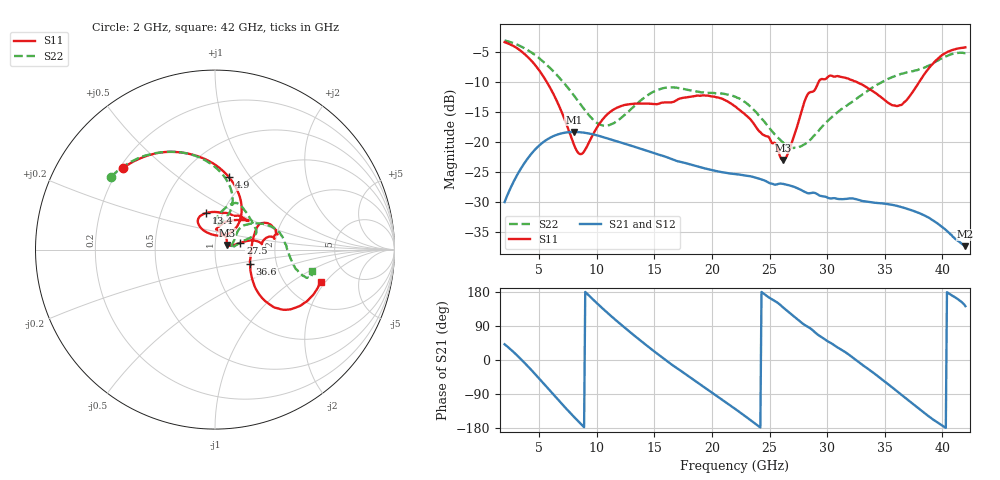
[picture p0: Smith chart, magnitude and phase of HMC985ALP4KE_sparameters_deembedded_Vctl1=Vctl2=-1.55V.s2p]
!s2p File: Measurements: S11, S21, S12, S22
# GHz S dB R 50.0
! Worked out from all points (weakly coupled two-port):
!   401 points, 2 GHz to 42 GHz, reference 50 ohm
!   highest |S21| = -18.30 dB at 8 GHz (marker M1); lowest = -37.4 dB at 42 GHz (marker M2)
!   lowest |S11| = -23.0 dB at 26.2 GHz (marker M3), VSWR 1.15, Z = 57 + j2.93 ohm
!   |S11| at or under -10 dB: 5.678 GHz to 29.25 GHz (23.57 GHz wide, 135 % of centre); 32.61 GHz to 37.97 GHz (5.359 GHz wide, 15.2 % of centre)
!   |S22| runs from -21.0 to -3.0 dB; largest |S21 - S12| = 0.00014
!   S11 on the Smith chart (normalised r, x): 2 GHz: 0.21, +0.36; 4.9 GHz: 0.82, +0.80; 13.4 GHz: 0.84, +0.36; 27.5 GHz: 1.33, +0.10; 36.6 GHz: 1.46, -0.24; 42 GHz: 3.08, -1.83
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2  -3.29 138.5  -30.03 41.5  -30.03 41.5  -3.01 145.0
3.4  -4.75 110.4  -24.48 2.7  -24.48 2.7  -3.98 121.8
4.9  -7.74 79.0  -20.75 -45.6  -20.76 -45.6  -5.82 98.1
6.2  -11.81 54.8  -19.03 -89.9  -19.04 -90.0  -8.10 80.6
8  -20.32 57.3  -18.30 -149.4  -18.31 -149.4  -12.16 68.4
8.7  -21.97 88.8  -18.38 -171.2  -18.39 -171.2  -13.97 69.5
10.8  -15.57 123.2  -19.30 127.9  -19.30 127.9  -17.25 88.6
13.4  -13.56 103.5  -20.86 61.0  -20.87 61.0  -13.72 82.0
15.4  -13.57 77.2  -22.11 13.3  -22.11 13.3  -11.19 68.9
18.9  -12.25 41.7  -24.16 -62.7  -24.16 -62.7  -11.61 42.8
22  -14.01 55.7  -25.35 -128.8  -25.35 -128.8  -12.41 20.5
24.5  -18.84 86.5  -26.38 175.0  -26.38 175.0  -16.47 15.6
26.2  -22.98 21.1  -27.00 138.2  -27.01 138.1  -20.13 6.8
27.5  -16.69 14.8  -27.79 105.1  -27.80 105.0  -20.86 7.9
28.2  -12.42 11.3  -28.48 89.5  -28.48 89.6  -20.17 15.3
28.7  -11.59 7.0  -28.47 79.8  -28.48 79.8  -19.27 21.3
31.1  -9.06 18.8  -29.54 29.7  -29.53 29.6  -14.70 40.8
33.3  -10.69 29.7  -29.93 -18.0  -29.94 -18.1  -11.75 34.1
35.4  -13.55 9.3  -30.42 -66.4  -30.43 -66.4  -9.37 22.0
36.6  -13.51 -22.1  -30.95 -95.4  -30.96 -95.4  -8.53 13.6
39.6  -6.08 -42.1  -33.63 -165.3  -33.62 -165.2  -6.38 -14.8
42  -4.16 -17.1  -37.40 142.2  -37.40 142.0  -5.11 -12.3
